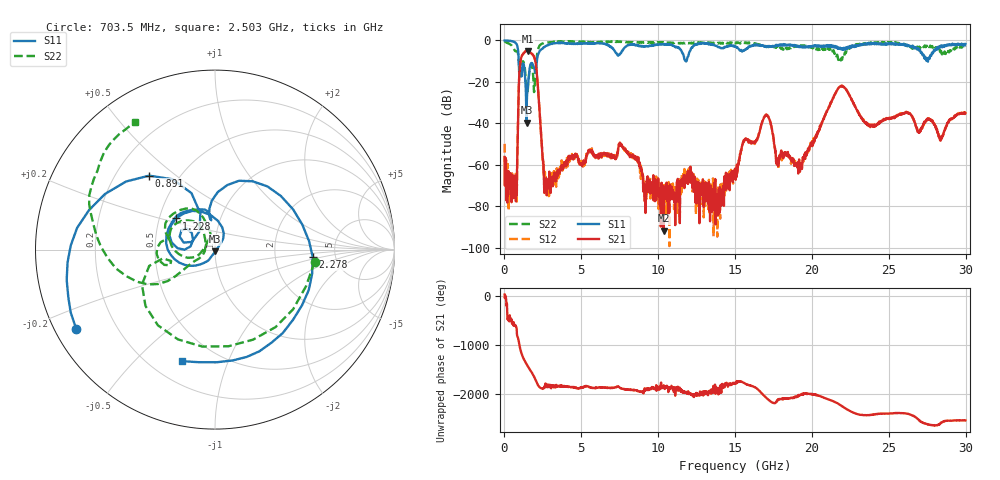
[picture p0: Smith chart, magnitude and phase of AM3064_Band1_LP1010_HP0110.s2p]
# Hz S DB R 50.0
!freq dBS11 angS11 dBS21 angS21 dBS12 angS12 dBS22 angS22
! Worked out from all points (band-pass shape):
!   1600 points, 10 MHz to 29.98 GHz, reference 50 ohm
!   highest |S21| = -5.02 dB at 1.51 GHz (marker M1); lowest = -91.8 dB at 10.36 GHz (marker M2)
!   |S21| within 3 dB of the highest: 1.101 GHz to 1.929 GHz (828.7 MHz wide, 54.7 % of centre)
!   lowest |S11| = -39.7 dB at 1.435 GHz (marker M3), VSWR 1.02, Z = 50.1 - j1.03 ohm
!   |S11| at or under -10 dB: 931.6 MHz to 2.107 GHz (1.176 GHz wide, 77.4 % of centre); 11.80536 GHz to 11.83947 GHz (34.11 MHz wide, 0.288 % of centre); 27.52359 GHz to 27.55058 GHz (26.99 MHz wide, 0.098 % of centre)
!   |S22| runs from -24.9 to -0.4 dB; largest |S21 - S12| = 0.0078
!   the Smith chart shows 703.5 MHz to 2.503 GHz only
!   S11 on the Smith chart (normalised r, x): 703.5 MHz: 0.06, -0.26; 891 MHz: 0.34, +0.40; 1.228 GHz: 0.61, +0.23; 2.278 GHz: 3.36, -0.41; 2.503 GHz: 0.32, -0.69
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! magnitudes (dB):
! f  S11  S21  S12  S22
! 10 MHz  0.0  -56.2  -49.9  -0.4
! 703.5 MHz  -1.0  -65.2  -67.8  -5.1
! 891 MHz  -5.2  -35.3  -35.4  -6.9
! 1.041 GHz  -13.3  -10.2  -10.1  -9.9
! 1.228 GHz  -11.1  -6.4  -6.4  -10.3
! 1.435 GHz  -39.7  -5.1  -5.0  -22.2
! 1.51 GHz  -23.4  -5.0  -5.0  -24.6
! 1.978 GHz  -14.8  -9.0  -9.1  -19.9
! 2.278 GHz  -5.2  -33.4  -33.4  -2.6
! 2.503 GHz  -3.8  -57.4  -57.0  -1.5
! 2.859 GHz  -2.2  -67.4  -70.3  -0.9
! 5.015 GHz  -1.5  -59.5  -58.7  -0.8
! 7.582 GHz  -6.1  -50.6  -50.6  -0.7
! 10 GHz  -2.0  -66.6  -72.5  -1.0
! 10.36 GHz  -2.0  -91.8  -72.1  -1.0
! 15 GHz  -3.1  -62.0  -63.2  -1.4
! 17.01 GHz  -3.2  -36.1  -36.1  -3.0
! 17.8 GHz  -2.2  -60.8  -57.6  -3.5
! 19.99 GHz  -3.0  -49.4  -50.1  -3.2
! 21.88 GHz  -4.1  -22.1  -22.2  -8.8
! 25 GHz  -1.4  -37.6  -37.4  -1.0
! 29.98 GHz  -1.7  -35.1  -35.3  -3.1
